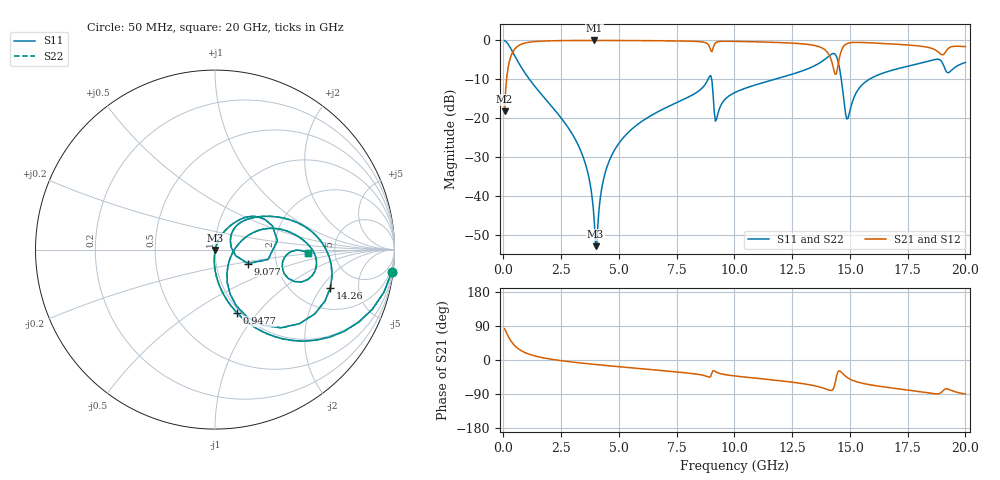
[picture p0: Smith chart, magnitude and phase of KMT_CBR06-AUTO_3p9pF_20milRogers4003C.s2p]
! Data measured by Modelithics Inc. support@modelithics.com 813-866-6335
! KEMET CBR06-AUTO 3.9pF, Pad Width= 0.851mm, Pad Length= 0.64mm, Pad Gap= 0.62mm, 20mil Rogers 4003C substrate Data, January 2022
# hz S ma R 50
! 2 Port Network Data from SP1.SP block
! freq  magS11  angS11  magS21  angS21  magS12  angS12  magS22  angS22
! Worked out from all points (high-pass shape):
!   401 points, 50 MHz to 20 GHz, reference 50 ohm
!   highest |S21| = -0.02 dB at 3.94 GHz (marker M1); lowest = -18.2 dB at 50 MHz (marker M2)
!   |S21| within 3 dB of the highest: 401.4 MHz to 14.02 GHz (13.61 GHz wide, 189 % of centre); 14.61 GHz to 18.83 GHz (4.222 GHz wide, 25.3 % of centre)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
!   lowest |S11| = -53.0 dB at 3.99 GHz (marker M3), VSWR 1.00, Z = 50.2 - j0.162 ohm
!   |S11| at or under -10 dB: 1.122 GHz to 8.861 GHz (7.738 GHz wide, 155 % of centre); 9.011 GHz to 11.76 GHz (2.747 GHz wide, 26.5 % of centre); 14.63 GHz to 15.84 GHz (1.219 GHz wide, 8 % of centre)
!   |S22| runs from -53.0 to -0.1 dB; largest |S21 - S12| = 0
!   S11 on the Smith chart (normalised r, x): 50 MHz: 1, -16; 947.8 MHz: 0.96, -0.79; 9.077 GHz: 1.43, -0.23; 14.26 GHz: 3.13, -2.46; 20 GHz: 3.15, -0.18
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5e7  0.9924 -7.2  0.1225 82.8  0.1225 82.8  0.9924 -7.2
3.4925e8  0.7546 -42.0  0.6553 47.9  0.6553 47.9  0.7546 -42.0
9.4775e8  0.3746 -70.7  0.9261 19.1  0.9261 19.1  0.3746 -70.7
3.391625e9  0.03509 -95.4  0.9975 -8.2  0.9975 -8.2  0.03509 -95.4
3.74075e9  0.01482 -93.4  0.998 -10.4  0.998 -10.4  0.01482 -93.4
3.94025e9  0.004303 -76.3  0.998 -11.6  0.998 -11.6  0.004303 -76.3
3.990125e9  0.00224 -46.1  0.998 -11.9  0.998 -11.9  0.00224 -46.1
4.33925e9  0.01655 69.3  0.9978 -14.0  0.9978 -14.0  0.01655 69.3
4.73825e9  0.03549 70.5  0.9972 -16.2  0.9972 -16.2  0.03549 70.5
6.73325e9  0.1226 61.6  0.9896 -27.2  0.9896 -27.2  0.1226 61.6
8.92775e9  0.3461 22.6  0.817 -45.3  0.817 -45.3  0.3461 22.6
9.077375e9  0.1995 -22.9  0.8008 -28.1  0.8008 -28.1  0.1995 -22.9
9.227e9  0.09691 28.1  0.9482 -32.3  0.9482 -32.3  0.09691 28.1
1.0025e10  0.2135 46.2  0.9706 -42.2  0.9706 -42.2  0.2135 46.2
1.336662e10  0.4559 21.0  0.871 -66.6  0.871 -66.6  0.4559 21.0
1.426438e10  0.6771 -18.3  0.4682 -77.9  0.4682 -77.9  0.6771 -18.3
1.451375e10  0.4978 -57.8  0.5342 -28.9  0.5342 -28.9  0.4978 -57.8
1.491275e10  0.09899 -11.5  0.9175 -47.3  0.9175 -47.3  0.09899 -11.5
1.551125e10  0.2646 23.8  0.9401 -61.0  0.9401 -61.0  0.2646 23.8
1.670825e10  0.403 15.5  0.9032 -72.9  0.9032 -72.9  0.403 15.5
1.90025e10  0.5162 -20.3  0.6506 -83.0  0.6506 -83.0  0.5162 -20.3
2e10  0.5193 -2.3  0.8313 -89.8  0.8313 -89.8  0.5193 -2.3
